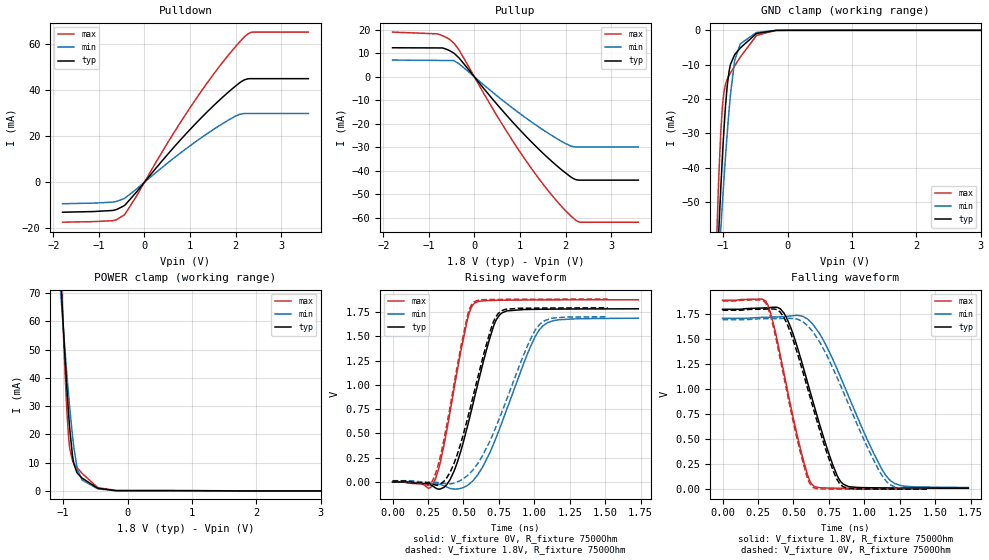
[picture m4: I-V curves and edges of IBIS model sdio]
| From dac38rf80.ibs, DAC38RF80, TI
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|   sdio Model
[Model]   sdio
Model_type   I/O
Polarity   Non-Inverting
Enable   Active-Low
Vinl = 0.54
Vinh = 1.26
Vmeas = 0.9
Vref = 0
Cref = 2pF
Rref = 100
|   typ   min   max
|   (nom PVT)   (fast PVT)   (slow PVT)
C_comp   2.866e-13   2.700e-13   3.018e-13
| Where nom  PVT is Nominal Process, 1.8V, 27C
|   Fast PVT is Strong Process,  1.89V, -40C
|   Slow PVT is Weak Process,   1.71V, 105C
[Model spec]
|subparameter
Vinl   0.54   0.51   0.57
Vinh   1.26   1.19   1.33
[Voltage Range]   1.8   1.71   1.89
|Junction Temperature
[Temperature Range]   27   105   -40
[Pullup Reference]   1.8   1.71   1.89
[Pulldown Reference]   0   0   0
[Power Clamp Reference]   1.8   1.71   1.89
[GND Clamp Reference]   0   0   0
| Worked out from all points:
|   slope of the pulldown table from 0 to 0.27 V, typ, clamps not added: 41.5 ohm
|   slope of the pullup table from 0 to 0.27 V, typ, clamps not added: 41.8 ohm
|   GND clamp passes 1 mA (typ) near -0.49 V on its own axis
|   POWER clamp passes 1 mA (typ) near -0.47 V on its own axis
|   falling waveform, V_fixture 1.8V, R_fixture 7500Ohm: 20-80 % time 224ps typ, 314ps min, 171ps max; typ from 1.8 V to 0.011 V
|   rising waveform, V_fixture 0V, R_fixture 7500Ohm: 20-80 % time 186ps typ, 264ps min, 141ps max; typ from 0 V to 1.78 V
|   rising waveform, V_fixture 1.8V, R_fixture 7500Ohm: 20-80 % time 191ps typ, 278ps min, 144ps max; typ from 0.01 V to 1.79 V
|   falling waveform, V_fixture 0V, R_fixture 7500Ohm: 20-80 % time 225ps typ, 319ps min, 171ps max; typ from 1.79 V to 0.001 V
[Pulldown]
|   Voltage   I(typ)   I(min)   I(max)
-1.8V     -12.98mA   -9.299mA   -17.31mA
-700.5mV  -12.23mA   -8.616mA   -16.66mA
-437.4mV  -10.01mA   -6.958mA   -13.99mA
-180mV    -4.338mA   -3.01mA    -6.13mA
554.9mV   13.14mA    9.096mA    18.59mA
1.114V    25.25mA    17.45mA    35.66mA
1.545V    33.75mA    23.29mA    47.61mA
1.976V    41.34mA    28.45mA    58.29mA
2.131V    43.71mA    29.66mA    61.73mA
2.277V    44.88mA    29.85mA    64.41mA
2.392V    44.94mA    29.85mA    65.14mA
3.6V      44.94mA    29.85mA    65.14mA
[GND Clamp]
|   Voltage   I(typ)   I(min)   I(max)
-1.8V     -418.3mA   -319.6mA   -575.1mA
-1.121V   -81.4mA    -84.1mA    -72.83mA
-1.074V   -61.09mA   -69.22mA   -46.11mA
-1.063V   -56.45mA   -65.74mA   -40.6mA
-1.035V   -45.24mA   -57.12mA   -28.89mA
-987.3mV  -28.86mA   -43.43mA   -17.99mA
-934.2mV  -15.78mA   -29.43mA   -14.13mA
-886.9mV  -10.02mA   -18.89mA   -12.43mA
-816.7mV  -6.995mA   -8.499mA   -10.26mA
-732.6mV  -5.114mA   -3.923mA   -7.764mA
-488.3mV  -1.028mA   -692.5uA   -1.66mA
3.6V      0A         0A         0A
[Pullup]
|   Voltage   I(typ)   I(min)   I(max)
-1.8V     12.39mA    7.162mA    19.07mA
-818.5mV  12.32mA    7.009mA    18.32mA
-698.4mV  12.3mA     6.99mA     17.49mA
-461.1mV  10.2mA     6.953mA    14.55mA
-342.8mV  8.128mA    5.586mA    11.55mA
564.4mV   -13.25mA   -9.156mA   -18.78mA
1.112V    -24.93mA   -17.25mA   -35.15mA
1.751V    -36.87mA   -25.58mA   -51.58mA
2.101V    -42.39mA   -29.31mA   -58.9mA
2.218V    -43.68mA   -29.79mA   -60.92mA
2.326V    -43.96mA   -29.81mA   -61.86mA
3.6V      -43.96mA   -29.81mA   -61.86mA
[POWER Clamp]
|   Voltage   I(typ)   I(min)   I(max)
-1.8V     456.8mA    335.7mA    653mA
-1.032V   72.98mA    68.15mA    78.03mA
-1.008V   62.5mA     60.65mA    62.92mA
-973.8mV  48.38mA    50.36mA    43.39mA
-938.2mV  34.89mA    40.14mA    26.74mA
-917.4mV  27.86mA    34.48mA    19.69mA
-894.7mV  21.14mA    28.65mA    14.64mA
-842.4mV  10.7mA     17.01mA    10.06mA
-774mV    6.111mA    7.393mA    7.94mA
-707.6mV  4.583mA    3.902mA    6.257mA
-469.4mV  1.026mA    830.1uA    1.318mA
3.6V      0A         0A         0A
[Ramp]
R_load = 7500
|   typ   min   max
dV/dt_r   1.07154/1.86394e-10   1.01552/2.64375e-10   1.12695/1.41572e-10
dV/dt_f   1.07159/2.24227e-10   1.01555/3.14263e-10   1.12698/1.71075e-10
[Falling Waveform]
V_fixture = 1.8V
V_fixture_min = 1.71V
V_fixture_max = 1.89V
R_fixture = 7500Ohm
|   Time   V(typ)   V(min)   V(max)
0s        1.796V     1.706V     1.885V
318.7ps   1.811V     1.716V     1.841V
406.7ps   1.802V     1.721V     1.342V
455ps     1.7V       1.725V     1.008V
571.1ps   1.208V     1.722V     284.1mV
640.3ps   862.7mV    1.639V     35.37mV
834ps     74.94mV    1.113V     10.62mV
1.066ns   14.59mV    358.1mV    9.174mV
1.181ns   13.22mV    90.55mV    8.862mV
1.734ns   11.19mV    17.19mV    8.018mV
[Rising Waveform]
V_fixture = 0V
V_fixture_min = 0V
V_fixture_max = 0V
R_fixture = 7500Ohm
|   Time   V(typ)   V(min)   V(max)
0s        87.83nV    326.2nV    91.32nV
290.1ps   -49.13mV   -17.6mV    -10.78mV
338.4ps   -71.34mV   -25.63mV   214.5mV
434ps     112.8mV    -72.78mV   961.2mV
531.3ps   590.8mV    -31.46mV   1.692V
579ps     875.3mV    34.47mV    1.842V
750.8ps   1.714V     533.8mV    1.872V
970.5ps   1.778V     1.387V     1.875V
1.061ns   1.78V      1.61V      1.876V
1.734ns   1.784V     1.688V     1.878V
[Rising Waveform]
V_fixture = 1.8V
V_fixture_min = 1.71V
V_fixture_max = 1.89V
R_fixture = 7500Ohm
|   Time   V(typ)   V(min)   V(max)
0s        9.681mV    13.25mV    7.188mV
290.1ps   -25.95mV   -2.876mV   37.48mV
347.6ps   -11.36mV   -9.124mV   332.2mV
434ps     193.3mV    -11.1mV    1.013V
527.7ps   648.1mV    65.3mV     1.71V
571.1ps   900.2mV    131.6mV    1.851V
683.7ps   1.527V     413mV      1.88V
742.3ps   1.731V     614.5mV    1.881V
1.041ns   1.792V     1.63V      1.884V
1.518ns   1.794V     1.703V     1.885V
[Falling Waveform]
V_fixture = 0V
V_fixture_min = 0V
V_fixture_max = 0V
R_fixture = 7500Ohm
|   Time   V(typ)   V(min)   V(max)
0s        1.786V     1.693V     1.878V
304.8ps   1.798V     1.702V     1.858V
359.5ps   1.799V     1.703V     1.611V
434ps     1.711V     1.704V     1.111V
547.4ps   1.264V     1.684V     375.7mV
628ps     866.1mV    1.587V     31.06mV
779.5ps   188.2mV    1.204V     2.199mV
849.4ps   26.22mV    978.2mV    1.864mV
1.16ns    1.8mV      71.03mV    1.316mV
1.442ns   1.344mV    2.3mV      1.027mV
